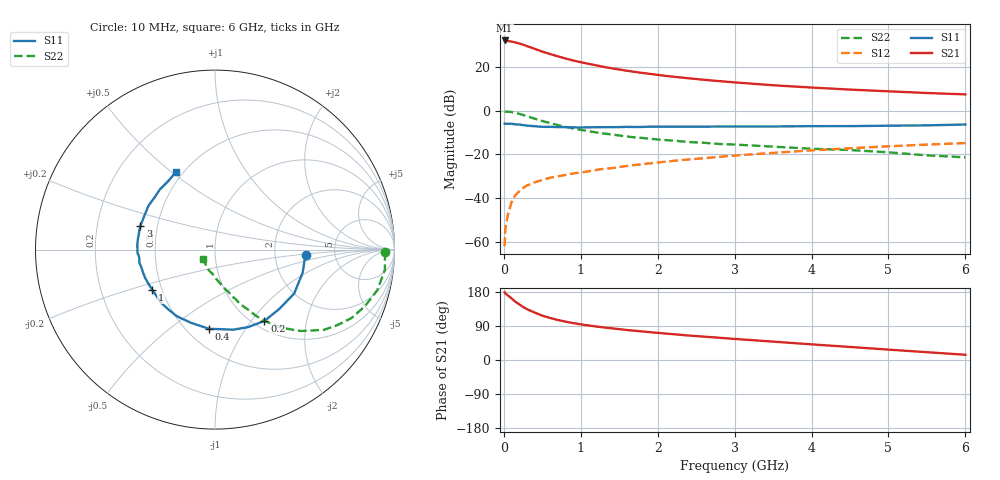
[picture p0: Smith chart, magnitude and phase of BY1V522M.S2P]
! SIEMENS Small Signal Semiconductors
! BFY420
! Si NPN RF SIEGET Grounded Emitter Transistor in MICRO-X
! VCE = 1.5 V  IC = 22 mA
! Common Emitter S-Parameters:  October  1996
# GHz  S  MA  R  50
!  f  S11  S21  S12  S22
! GHz  MAG  ANG  MAG  ANG  MAG  ANG  MAG  ANG
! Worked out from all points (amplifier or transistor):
!   36 points, 10 MHz to 6 GHz, reference 50 ohm
!   highest |S21| = 32.1 dB at 10 MHz (marker M1)
!   |S21| within 3 dB of that: start of sweep to 334.5 MHz
!   unconditionally stable (mu >= 1): start of sweep to 10.31 MHz; 1.763 GHz to end of sweep
!   at 250 MHz: K = 0.32, MSG = 32.8 dB, |S12| = -35.3 dB
!   at 1.4 GHz: K = 0.94, MSG = 22.8 dB, |S12| = -26.3 dB
!   at 6 GHz: K = 1.08, MAG = 9.4 dB, |S12| = -14.8 dB
!   S11 on the Smith chart (normalised r, x): 10 MHz: 3.04, -0.25; 200 MHz: 1.12, -1.16; 400 MHz: 0.64, -0.70; 1 GHz: 0.44, -0.24; 3 GHz: 0.40, +0.13; 6 GHz: 0.46, +0.52
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0.01  0.5084 -3.5  40.45 178.7  0.0008 101.9  0.9488 -0.8
0.02  0.5024 -6.6  40.28 175.7  0.002 82.1  0.9475 -2.2
0.05  0.5051 -14.7  39.22 170.6  0.004 83.4  0.9533 -6.7
0.1  0.5046 -29.0  38.25 162.7  0.0081 78.4  0.9323 -14.0
0.15  0.4876 -42.5  36.37 153.7  0.0118 73.9  0.8927 -20.7
0.2  0.4837 -55.3  34.53 147.0  0.0143 71.0  0.8511 -26.6
0.25  0.4695 -66.9  32.26 140.0  0.0171 66.2  0.7991 -31.9
0.3  0.4574 -77.3  30.08 134.3  0.0195 64.3  0.7532 -36.4
0.4  0.4424 -94.3  26.09 125.2  0.023 60.9  0.6591 -43.5
0.5  0.4291 -108.2  22.47 117.0  0.0261 58.9  0.5829 -48.7
0.6  0.4278 -119.7  19.82 111.0  0.0293 57.5  0.5207 -52.8
0.7  0.4227 -128.1  17.59 105.7  0.0316 56.6  0.471 -56.0
0.8  0.4224 -136.1  15.67 101.3  0.034 55.8  0.4274 -58.6
1  0.4149 -147.2  12.85 94.1  0.0386 56.3  0.3656 -62.4
1.1  0.4168 -152.8  11.83 91.1  0.0413 57.2  0.3414 -64.5
1.6  0.4276 -170.1  8.209 79.1  0.0545 56.4  0.2577 -71.5
2.2  0.4338 176.4  5.998 68.1  0.0713 54.8  0.2075 -78.4
3  0.4363 162.4  4.45 55.6  0.0945 50.3  0.1688 -86.3
3.5  0.4365 154.0  3.826 48.5  0.1088 47.1  0.1509 -91.5
4.5  0.4447 139.3  3.045 34.4  0.1387 38.5  0.1263 -102.1
5.5  0.4629 123.8  2.542 20.6  0.1683 29.0  0.0954 -124.7
6  0.4844 116.7  2.367 13.8  0.1821 24.0  0.0861 -142.5
